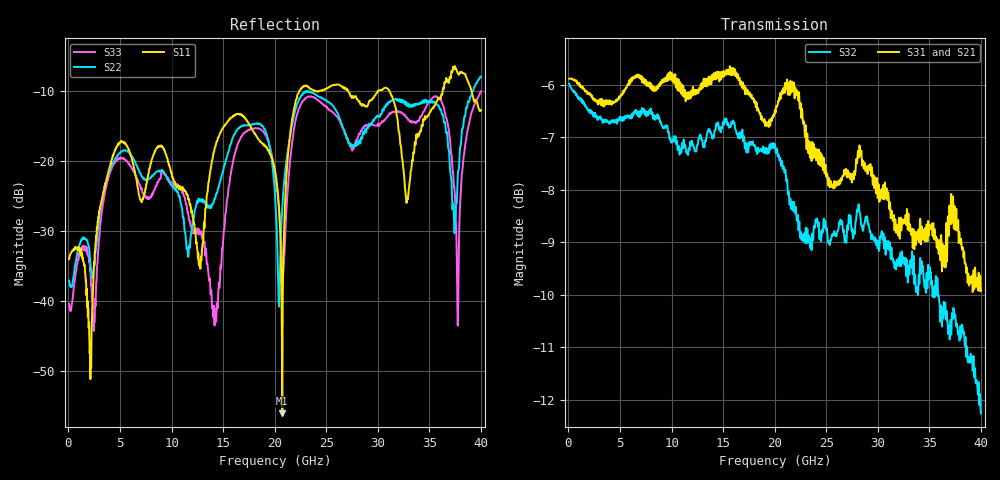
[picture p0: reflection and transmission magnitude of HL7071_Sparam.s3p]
! Created Mon Feb 28 12:57:26 2022
# hz S ma R 50
! 3 Port Network Data from SP2.SP block
! freq  magS11  angS11  magS12  angS12  magS13  angS13
!  magS21  angS21
!  magS22  angS22  magS23  angS23
!  magS31  angS31  magS32  angS32
!  magS33  angS33
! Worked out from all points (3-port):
!   2000 points, 70 MHz to 40 GHz, reference 50 ohm
!   strongest paths, dB at 70 MHz, 10.06 GHz, 20.04 GHz, 30.03 GHz, 40 GHz:
!     S31: -5.9, -5.8, -6.5, -8.1, -9.9
!     S21: -5.8, -5.8, -6.6, -8.0, -10.3
!     S32: -6.0, -7.1, -7.2, -9.0, -12.3
!   lowest |S11| = -56.1 dB at 20.74 GHz (marker M1), VSWR 1.00, Z = 50.1 - j0.0928 ohm
!   |S11| at or under -10 dB: start of sweep to 22.42 GHz; 27.12 GHz to 30.03 GHz (2.909 GHz wide, 10.2 % of centre); 31.13 GHz to 36.3 GHz (5.173 GHz wide, 15.3 % of centre)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
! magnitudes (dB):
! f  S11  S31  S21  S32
! 70 MHz  -34.0  -5.9  -5.8  -6.0
! 2.147 GHz  -51.0  -6.2  -6.1  -6.5
! 4.764 GHz  -17.8  -6.3  -6.2  -6.7
! 14.17 GHz  -18.2  -5.9  -6.0  -6.9
! 20.04 GHz  -21.6  -6.5  -6.6  -7.2
! 20.74 GHz  -56.1  -6.1  -6.4  -7.5
! 22.72 GHz  -9.4  -6.7  -6.6  -8.9
! 35.95 GHz  -11.2  -9.2  -9.2  -10.1
! 37.74 GHz  -7.5  -8.7  -8.7  -10.7
! 40 GHz  -12.8  -9.9  -10.3  -12.3
